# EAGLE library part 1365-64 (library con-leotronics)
DUAL ROW STRAIGHT HEADER 1364 SERIES. 1.27mm x 1.27mm. Without Fixing Post. SMT Source: http://www.leotronics.co.uk/Conexcon/Data%20Sheets/sec.%20A/1364ing.pdf
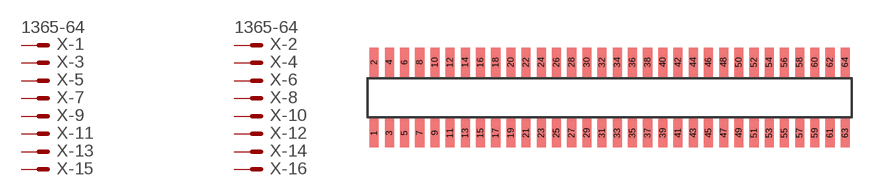
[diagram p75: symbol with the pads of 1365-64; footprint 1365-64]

Designator prefix X; gates -1=MVAL -2=MVAL -3=M -4=M -5=M -6=M -7=M -8=M -9=M -10=M -11=M -12=M -13=M -14=M -15=M -16=M -17=M -18=M -19=M -20=M -21=M -22=M -23=M -24=M -25=M -26=M -27=M -28=M -29=M -30=M -31=M -32=M -33=M -34=M -35=M -36=M -37=M -38=M -39=M -40=M -41=M -42=M -43=M -44=M -45=M -46=M -47=M -48=M -49=M -50=M -51=M -52=M -53=M -54=M -55=M -56=M -57=M -58=M -59=M -60=M -61=M -62=M -63=M -64=M

## 1365-64 (OC_FARNELL: unknown; OC_NEWARK: unknown)  [1365-64]
1  -1:S  pas
2  -2:S  pas
3  -3:S  pas
4  -4:S  pas
5  -5:S  pas
6  -6:S  pas
7  -7:S  pas
8  -8:S  pas
9  -9:S  pas
10  -10:S  pas
11  -11:S  pas
12  -12:S  pas
13  -13:S  pas
14  -14:S  pas
15  -15:S  pas
16  -16:S  pas
17  -17:S  pas
18  -18:S  pas
19  -19:S  pas
20  -20:S  pas
21  -21:S  pas
22  -22:S  pas
23  -23:S  pas
24  -24:S  pas
25  -25:S  pas
26  -26:S  pas
27  -27:S  pas
28  -28:S  pas
29  -29:S  pas
30  -30:S  pas
31  -31:S  pas
32  -32:S  pas
33  -33:S  pas
34  -34:S  pas
35  -35:S  pas
36  -36:S  pas
37  -37:S  pas
38  -38:S  pas
39  -39:S  pas
40  -40:S  pas
41  -41:S  pas
42  -42:S  pas
43  -43:S  pas
44  -44:S  pas
45  -45:S  pas
46  -46:S  pas
47  -47:S  pas
48  -48:S  pas
49  -49:S  pas
50  -50:S  pas
51  -51:S  pas
52  -52:S  pas
53  -53:S  pas
54  -54:S  pas
55  -55:S  pas
56  -56:S  pas
57  -57:S  pas
58  -58:S  pas
59  -59:S  pas
60  -60:S  pas
61  -61:S  pas
62  -62:S  pas
63  -63:S  pas
64  -64:S  pas

## Footprint 1365-64 (pad centres in mm)
DUAL ROW STRAIGHT HEADER 1364 SERIES. 1.27mm x 1.27mm. Without Fixing Post. SMT Source: http://www.leotronics.co.uk/Conexcon/Data%20Sheets/sec.%20A/1364ing.pdf
smd 0.76 x 2.4: 1 -19.685,-2.95; 2 -19.685,2.95; 3 -18.415,-2.95; 4 -18.415,2.95; 5 -17.145,-2.95; 6 -17.145,2.95; 7 -15.875,-2.95; 8 -15.875,2.95; 9 -14.605,-2.95; 10 -14.605,2.95; 11 -13.335,-2.95; 12 -13.335,2.95; 13 -12.065,-2.95; 14 -12.065,2.95; 15 -10.795,-2.95; 16 -10.795,2.95; 17 -9.525,-2.95; 18 -9.525,2.95; 19 -8.255,-2.95; 20 -8.255,2.95; 21 -6.985,-2.95; 22 -6.985,2.95; 23 -5.715,-2.95; 24 -5.715,2.95; 25 -4.445,-2.95; 26 -4.445,2.95; 27 -3.175,-2.95; 28 -3.175,2.95; 29 -1.905,-2.95; 30 -1.905,2.95; 31 -0.635,-2.95; 32 -0.635,2.95; 33 0.635,-2.95; 34 0.635,2.95; 35 1.905,-2.95; 36 1.905,2.95; 37 3.175,-2.95; 38 3.175,2.95; 39 4.445,-2.95; 40 4.445,2.95; 41 5.715,-2.95; 42 5.715,2.95; 43 6.985,-2.95; 44 6.985,2.95; 45 8.255,-2.95; 46 8.255,2.95; 47 9.525,-2.95; 48 9.525,2.95; 49 10.795,-2.95; 50 10.795,2.95; 51 12.065,-2.95; 52 12.065,2.95; 53 13.335,-2.95; 54 13.335,2.95; 55 14.605,-2.95; 56 14.605,2.95; 57 15.875,-2.95; 58 15.875,2.95; 59 17.145,-2.95; 60 17.145,2.95; 61 18.415,-2.95; 62 18.415,2.95; 63 19.685,-2.95; 64 19.685,2.95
